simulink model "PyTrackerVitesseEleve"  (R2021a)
settings: Solver=ode15s  StartTime=0.0  StopTime=5  RelTol=1e-3  EnableMultiTasking=on
libraries: fl_lib x20, nesl_utility x7

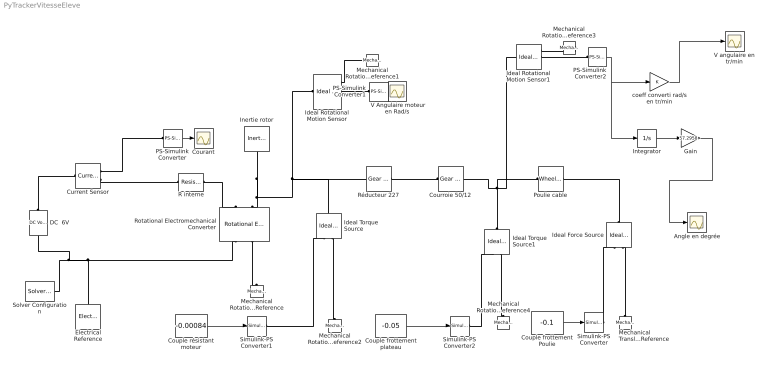
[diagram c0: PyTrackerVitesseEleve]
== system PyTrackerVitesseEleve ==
  " V Angulaire moteur en Rad/s" : Scope
  Angle en degrée : Scope
  Couple frottement Poulie : Constant  Value=-0.1
  Couple frottement plateau : Constant  Value=-0.05
  Couple résistant moteur : Constant  Value=-0.00084
  Courant : Scope
  Courroie 50/12 : fl_lib/Mechanical/Mechanisms/Gear Box  ratio=20  t_in_specify=off  t_in_priority=None  t_in=0 N*m  t_in_nominal_specify=off  t_in_nominal_unit=N*m  t_in_nominal_value=1  t_out_specify=off  t_out_priority=None  t_out=0 N*m  t_out_nominal_specify=off  t_out_nominal_unit=N*m  t_out_nominal_value=1
  Current Sensor : fl_lib/Electrical/Electrical Sensors/Current Sensor
  DC  6V : fl_lib/Electrical/Electrical Sources/DC Voltage Source  v0=10 V
  Electrical Reference : fl_lib/Electrical/Electrical Elements/Electrical Reference
  Gain : Gain  Gain=57.2958
  Ideal Force Source : fl_lib/Mechanical/Mechanical Sources/Ideal Force Source
  Ideal Rotational Motion Sensor : fl_lib/Mechanical/Mechanical Sensors/Ideal Rotational Motion Sensor  wrap_angle=simscape.enum.onoff.on  offset=0 rev
  Ideal Rotational Motion Sensor1 : fl_lib/Mechanical/Mechanical Sensors/Ideal Rotational Motion Sensor  wrap_angle=simscape.enum.onoff.off  offset=0 rev
  Ideal Torque Source : fl_lib/Mechanical/Mechanical Sources/Ideal Torque Source
  Ideal Torque Source1 : fl_lib/Mechanical/Mechanical Sources/Ideal Torque Source
  Inertie rotor : fl_lib/Mechanical/Rotational Elements/Inertia  inertia=0.0000006 kg*m^2  num_ports=foundation.enum.numPorts2.one  w_specify=on  w_priority=High  w=0 rad/s  w_nominal_specify=off  w_nominal_unit=rad/s  w_nominal_value=1  t_specify=off  t_priority=None  t=0 N*m  t_nominal_specify=off  t_nominal_unit=N*m  t_nominal_value=1
  Integrator : Integrator
  Mechanical Rotational Reference{,1..4} (5 alike) : fl_lib/Mechanical/Rotational Elements/Mechanical Rotational Reference
  Mechanical Translational Reference : fl_lib/Mechanical/Translational Elements/Mechanical Translational Reference
  PS-Simulink Converter : nesl_utility/PS-Simulink Converter  PhysicalDomain=network_engine_domain  SubClassName=ps_output  LeftPortType=input  RightPortType=output  PseudoPeriodic=off  Frequencies=[]  Unit=A  AffineConversion=off
  PS-Simulink Converter1 : nesl_utility/PS-Simulink Converter  PhysicalDomain=network_engine_domain  SubClassName=ps_output  LeftPortType=input  RightPortType=output  PseudoPeriodic=off  Frequencies=[]  Unit=1  AffineConversion=off
  PS-Simulink Converter2 : nesl_utility/PS-Simulink Converter  PhysicalDomain=network_engine_domain  SubClassName=ps_output  LeftPortType=input  RightPortType=output  PseudoPeriodic=off  Frequencies=[]  Unit=1  AffineConversion=off
  Poulie cable : fl_lib/Mechanical/Mechanisms/Wheel and Axle  R=0.15 m  or=1  t_specify=off  t_priority=None  t=0 N*m  t_nominal_specify=off  t_nominal_unit=N*m  t_nominal_value=1  f_specify=off  f_priority=None  f=0 N  f_nominal_specify=off  f_nominal_unit=N  f_nominal_value=1
  R interne : fl_lib/Electrical/Electrical Elements/Resistor  R=4.2 Ohm  i_specify=off  i_priority=None  i=0 A  i_nominal_specify=off  i_nominal_unit=A  i_nominal_value=1  v_specify=off  v_priority=None  v=0 V  v_nominal_specify=off  v_nominal_unit=V  v_nominal_value=1
  Rotational Electromechanical Converter : fl_lib/Electrical/Electrical Elements/Rotational Electromechanical Converter  K=0.014 V/(rad/s)  i_specify=off  i_priority=None  i=0 A  i_nominal_specify=off  i_nominal_unit=A  i_nominal_value=1  v_specify=off  v_priority=None  v=0 V  v_nominal_specify=off  v_nominal_unit=V  v_nominal_value=1  t_specify=off  t_priority=None  t=0 N*m  t_nominal_specify=off  t_nominal_unit=N*m  t_nominal_value=1  w_specify=off  w_priority=High  w=0 rpm  w_nominal_specify=off  w_nominal_unit=rad/s  w_nominal_value=1
  Réducteur 227 : fl_lib/Mechanical/Mechanisms/Gear Box  ratio=20  t_in_specify=off  t_in_priority=None  t_in=0 N*m  t_in_nominal_specify=off  t_in_nominal_unit=N*m  t_in_nominal_value=1  t_out_specify=off  t_out_priority=None  t_out=0 N*m  t_out_nominal_specify=off  t_out_nominal_unit=N*m  t_out_nominal_value=1
  Simulink-PS Converter : nesl_utility/Simulink-PS Converter  PhysicalDomain=network_engine_domain  SubClassName=ps_input  LeftPortType=input  RightPortType=output  PseudoPeriodic=off  Frequencies=[]  NoiseDistribution=none  NoiseParameters=[]  Unit=1  AffineConversion=off  FilteringAndDerivatives=zero  SimscapeFilterOrder=1  InputFilterTimeConstant=.001  UdotUserProvided=0
  Simulink-PS Converter1 : nesl_utility/Simulink-PS Converter  PhysicalDomain=network_engine_domain  SubClassName=ps_input  LeftPortType=input  RightPortType=output  PseudoPeriodic=off  Frequencies=[]  NoiseDistribution=none  NoiseParameters=[]  Unit=1  AffineConversion=off  FilteringAndDerivatives=zero  SimscapeFilterOrder=1  InputFilterTimeConstant=.001  UdotUserProvided=0
  Simulink-PS Converter2 : nesl_utility/Simulink-PS Converter  PhysicalDomain=network_engine_domain  SubClassName=ps_input  LeftPortType=input  RightPortType=output  PseudoPeriodic=off  Frequencies=[]  NoiseDistribution=none  NoiseParameters=[]  Unit=1  AffineConversion=off  FilteringAndDerivatives=zero  SimscapeFilterOrder=1  InputFilterTimeConstant=.001  UdotUserProvided=0
  Solver Configuration : nesl_utility/Solver Configuration  PhysicalDomain=network_engine_domain  SubClassName=solver  LeftPortType=input  RightPortType=generic  Tones=[]  Harmonics=[]  SimulateNoise=off  Profile=off  UseLocalSampling=off  EnableSwitchedLinearOptims=on  FrequencyDomain=off  UseCCode=off  RelTol=0.001  AbsTol=1e-06  MinStep=1e-09  ToWorkspace=off  RevertToSquareIcSolve=off  NumHomotopyIterations=100  PhasorMode=off  PhasorModeNumHarmonics=1  DoDC=off  ResidualTolerance=1e-9  UseLocalSolver=off  LocalSolverChoice=NE_BACKWARD_EULER_ADVANCER  LocalSolverSampleTime=.001  DoFixedCost=off  MaxNonlinIter=3  MaxModeIter=2  ComputeImpulses=off  ImpulseIterations=2  LinearAlgebra=Sparse  EquationFormulation=NE_TIME_EF  DelaysMemoryBudget=1024  AutomaticFiltering=on  FilteringTimeConstant=0.001  PartitionStorageMethod=AS_NEEDED  PartitionMemoryBudget=1024  PartitionMethod=FAST
  V angulaire en tr/min : Scope
  coeff converti rad/s en tr/min : Gain
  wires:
  PS-Simulink Converter/1 -> Courant/1
  PS-Simulink Converter1/1 -> " V Angulaire moteur en Rad/s"/1
  Couple frottement Poulie/1 -> Simulink-PS Converter/1
  Couple résistant moteur/1 -> Simulink-PS Converter1/1
  Couple frottement plateau/1 -> Simulink-PS Converter2/1
  PS-Simulink Converter2/1 -> Integrator/1, coeff converti rad/s en tr/min/1
  Integrator/1 -> Gain/1
  Gain/1 -> Angle en degrée/1
  coeff converti rad/s en tr/min/1 -> V angulaire en tr/min/1
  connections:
  Current Sensor/RConn2 -- R interne/LConn1
  R interne/RConn1 -- Rotational Electromechanical Converter/LConn1
  DC  6V/RConn1 -- Solver Configuration/RConn1 -- Rotational Electromechanical Converter/RConn1 -- Electrical Reference/LConn1
  Rotational Electromechanical Converter/LConn2 -- Réducteur 227/LConn1 -- Ideal Torque Source/LConn1 -- Ideal Rotational Motion Sensor/LConn1 -- Inertie rotor/LConn1
  PS-Simulink Converter1/LConn1 -- Ideal Rotational Motion Sensor/RConn2
  Ideal Torque Source1/LConn1 -- Poulie cable/LConn1 -- Ideal Rotational Motion Sensor1/LConn1 -- Courroie 50/12/RConn1
  Ideal Force Source/LConn1 -- Poulie cable/RConn1
  Ideal Rotational Motion Sensor/RConn1 -- Mechanical Rotational Reference1/LConn1
  Mechanical Translational Reference/LConn1 -- Ideal Force Source/RConn2
  Simulink-PS Converter/RConn1 -- Ideal Force Source/RConn1
  Rotational Electromechanical Converter/RConn2 -- Mechanical Rotational Reference/LConn1
  DC  6V/LConn1 -- Current Sensor/LConn1
  Simulink-PS Converter1/RConn1 -- Ideal Torque Source/RConn1
  Ideal Torque Source/RConn2 -- Mechanical Rotational Reference2/LConn1
  Ideal Torque Source1/RConn2 -- Mechanical Rotational Reference4/LConn1
  Simulink-PS Converter2/RConn1 -- Ideal Torque Source1/RConn1
  Courroie 50/12/LConn1 -- Réducteur 227/RConn1
  Current Sensor/RConn1 -- PS-Simulink Converter/LConn1
  Mechanical Rotational Reference3/LConn1 -- Ideal Rotational Motion Sensor1/RConn1
  Ideal Rotational Motion Sensor1/RConn2 -- PS-Simulink Converter2/LConn1
